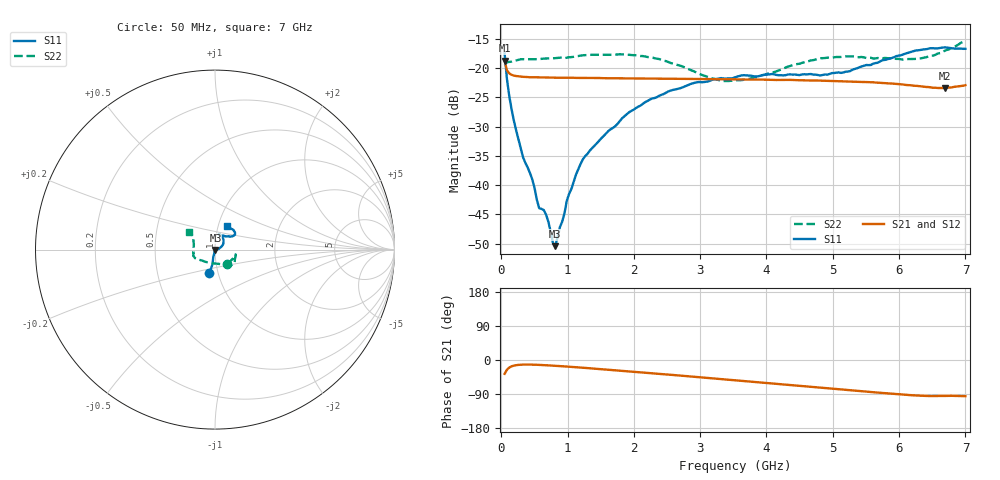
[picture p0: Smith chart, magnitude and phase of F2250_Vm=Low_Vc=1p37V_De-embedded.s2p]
! Integrated Device Technology
! Corporate Headquarters
! 6024 Silver Creek Valley Road
! San Jose, CA 95138  USA
! Phone:  1-408-284-8200
! Toll Free:  1-800-223-1366
! Webpage:  http://www.idt.com/
! Timing and RF Division
! 515 Groton Road, Suite 102
! Westford, MA 01886-6024
! Device:  F2250
! Description: Voltage Variable RF Attenuator
! Frequency:  50.0 -  6000.00 MHz
! Package:  3x3 mm Thin QFN Plastic Package: 16 pin
! Ports:  2 RF, 3 DC
!  Pin  1  = GND
!  Pin  2  = NC
!  Pin  3  = RF1  = Port 1
!  Pin  4  = NC
!  Pin  5  = GND
!  Pin  6  = GND
!  Pin  7  = GND
!  Pin  8  = GND
!  Pin  9  = NC
!  Pin 10  = RF2  = Port 2
!  Pin 11  = NC
!  Pin 12  = GND
!  Pin 13  = GND
!  Pin 14  = VCNTRL
!  Pin 15  = VDD
!  Pin 16  = VMODE
! Vcntrl:  1.370 Volts
! Vmode:  +0.000 Volts
! Vdd:  +3.30  Volts
! Current:  1.193 mA
! Data:  The device was measured on a the F2250 evaluation board which has
!  individual transmission lines to the RF pins.  Data was collected
!  using a calibrated network analyzer.  The evaluation board was
!  de-embedded using a TRL calibration technique.
!  The reference plane is the edge of the package pin.
! Misc:  SN 10
!  Action Tracker AT0258
! Date Measured:  2014-11-26
! Date:  2015-10-15  MJV
! Note:
!  Integrated Device Technology supplies this data as a sample of measured
!  data at the package pin for this product.  Your particular data for this
!  product may vary.
!  Data was taken at 25 degrees C.
!  Integrated Device Technology reserves the right to change this data at anytime.
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# GHz S dB R 50
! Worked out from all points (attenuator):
!   201 points, 50 MHz to 7 GHz, reference 50 ohm
!   highest |S21| = -18.75 dB at 50 MHz (marker M1); lowest = -23.4 dB at 6.687 GHz (marker M2)
!   lowest |S11| = -50.4 dB at 814.5 MHz (marker M3), VSWR 1.01, Z = 50.2 - j0.193 ohm
!   |S11| at or under -10 dB: start of sweep to end of sweep
!   |S22| runs from -22.2 to -15.3 dB; largest |S21 - S12| = 0.0003
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0.05  -17.49 -103.4  -18.75 -36.5  -18.74 -36.5  -19.47 -50.1
0.08475  -21.82 -99.4  -20.36 -25.7  -20.35 -25.7  -19.01 -26.1
0.1195  -24.74 -100.9  -20.89 -20.0  -20.90 -20.0  -18.95 -18.6
0.189  -28.95 -102.8  -21.28 -14.9  -21.27 -14.9  -18.77 -14.4
0.29325  -33.75 -99.7  -21.46 -12.4  -21.46 -12.4  -18.49 -13.9
0.467  -39.02 -104.7  -21.56 -12.2  -21.54 -12.2  -18.49 -14.6
0.57125  -43.93 -95.4  -21.58 -12.9  -21.57 -12.9  -18.46 -17.1
0.6755  -45.04 -79.7  -21.61 -13.8  -21.61 -13.8  -18.36 -19.3
0.77975  -49.92 -53.1  -21.62 -14.9  -21.62 -14.9  -18.32 -21.7
0.8145  -50.43 -39.8  -21.63 -15.3  -21.64 -15.3  -18.30 -22.7
0.98825  -42.66 -18.7  -21.64 -17.3  -21.65 -17.3  -18.21 -26.4
1.2315  -35.56 5.3  -21.68 -20.4  -21.68 -20.4  -17.81 -30.9
1.9265  -27.56 26.5  -21.76 -30.0  -21.76 -30.0  -17.72 -39.9
2.37825  -24.75 36.4  -21.80 -36.5  -21.80 -36.5  -18.45 -46.5
2.93425  -22.46 52.3  -21.85 -44.6  -21.85 -44.6  -20.71 -62.6
3.525  -21.58 67.3  -21.92 -53.4  -21.93 -53.4  -22.09 -101.6
4.7065  -21.11 69.7  -22.11 -71.2  -22.10 -71.3  -18.64 -155.4
5.22775  -20.60 53.2  -22.27 -79.2  -22.28 -79.2  -18.00 -163.9
5.85325  -18.38 37.7  -22.61 -88.6  -22.61 -88.7  -18.34 -175.9
6.33975  -16.86 39.1  -23.13 -94.4  -23.13 -94.4  -18.31 165.9
6.68725  -16.46 47.4  -23.41 -94.8  -23.40 -94.9  -17.03 150.5
7  -16.71 62.7  -22.92 -95.4  -22.93 -95.5  -15.28 146.2
